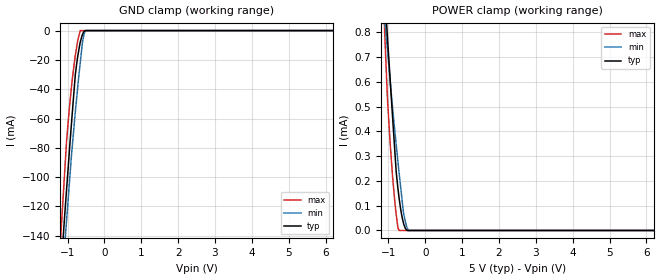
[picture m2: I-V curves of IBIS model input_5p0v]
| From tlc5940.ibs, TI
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|   input_5p0v Model
[Model]   input_5p0v
Model_type   Input
Vinl = 1.0
Vinh = 4.0
|   typ   min   max
|   (nom PVT)   (Fast PVT)   (slow PVT)
|Average
C_comp   1.262e-12   1.156e-12   1.274e-12
[Model Spec]
Vinl   1.0   0.9   1.1
Vinh   4.0   3.6   4.4
[Voltage Range]   5   4.5   5.5
|Ambient Temperature   25   85   -40
|Junction Temperature
[Temperature Range]   65   125   -40
[Power Clamp Reference]   5   4.5   5.5
[GND Clamp Reference]   0   0   0
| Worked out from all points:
|   GND clamp passes 1 mA (typ) near -0.56 V on its own axis
|   POWER clamp passes 1 mA (typ) near -1.12 V on its own axis
[GND Clamp]
|   Voltage   I(typ)   I(min)   I(max)
-5V       -1.796A    -1.693A    -1.901A
-1.245V   -189mA     -205.4mA   -166mA
-1.094V   -132.3mA   -152.5mA   -103.5mA
-1.029V   -109.6mA   -130.7mA   -76.55mA
-891.5mV  -62.96mA   -84.75mA   -38.05mA
-790mV    -30.56mA   -55.89mA   -17.3mA
-721mV    -17.35mA   -38.08mA   -6.651mA
-650mV    -7.456mA   -20.77mA   0A
-594.5mV  -2.762mA   -7.944mA   0A
-554mV    -631.2uA   -2.674mA   0A
-484.5mV  0A         0A         0A
10V       0A         0A         0A
[POWER Clamp]
|   Voltage   I(typ)   I(min)   I(max)
-5V       11.14mA    7.872mA    15.85mA
-1.177V   1.153mA    987uA      1.076mA
-1.085V   921.1uA    827uA      743.8uA
-1.04V    813.5uA    750.8uA    582.1uA
-957.5mV  620.4uA    612.6uA    364.2uA
-886mV    457uA      493.8uA    216.4uA
-790mV    240.8uA    349uA      66.93uA
-711.5mV  132.8uA    235.2uA    0A
-590mV    29.24uA    71.89uA    0A
-504.5mV  2.09uA     15.46uA    0A
-446mV    0A         0A         0A
10V       0A         0A         0A
